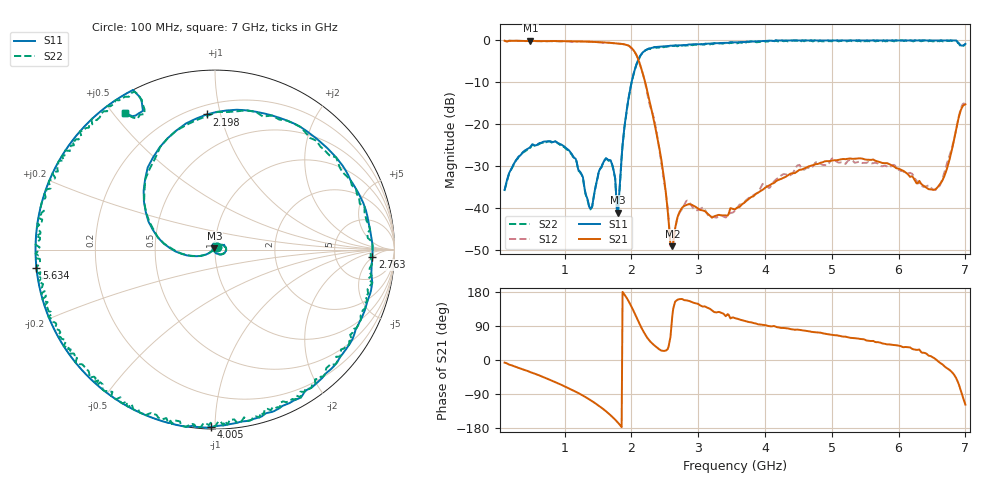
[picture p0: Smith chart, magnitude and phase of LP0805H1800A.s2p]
!	AVX	THIN	FILM	OPERATION
!	LP0805	High	Performance	Low	Pass	Filter	P/N	LP0805H1800ASTR
!	November	"13,"	2016
!Instrument:	"HEWLETT PACKARD,8720ES,US39172150,7.62 "
#	MHz	S	dB	R	50
!	Frq	S11(dB)	S11(deg)	S21(dB)	S21(deg)	S12(dB)	S12(deg)	S22(dB)	S22(deg)
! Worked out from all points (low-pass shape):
!   501 points, 100 MHz to 7 GHz, reference 50 ohm
!   highest |S21| = -0.04 dB at 486.4 MHz (marker M1); lowest = -49.2 dB at 2.612 GHz (marker M2)
!   |S21| within 3 dB of the highest: start of sweep to 2.06 GHz
!   lowest |S11| = -41.1 dB at 1.797 GHz (marker M3), VSWR 1.02, Z = 49.6 + j0.788 ohm
!   |S11| at or under -10 dB: start of sweep to 2.001 GHz
!   |S22| runs from -41.2 to 0.0 dB; largest |S21 - S12| = 0.063
!   S11 on the Smith chart (normalised r, x): 100 MHz: 1.02, +0.03; 2.198 GHz: 0.26, +0.91; 2.763 GHz: 14, -5; 4.005 GHz: 0.01, -0.98; 5.634 GHz: 0.00, -0.05; 7 GHz: 0.06, +0.54
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100  -35.75 54.8  -0.06 -6.9  -0.08 -6.6  -35.75 54.8
486.4  -25.42 26.5  -0.04 -32.1  -0.04 -31.5  -25.62 26.3
969.4  -25.07 -20.7  -0.17 -67.2  -0.22 -66.5  -25.07 -20.8
1259.2  -32.23 -66.5  -0.27 -92.6  -0.25 -92.4  -32.23 -66.6
1383.4  -40.19 -140.5  -0.30 -105.7  -0.34 -105.5  -40.39 -140.6
1535.2  -30.58 115.4  -0.42 -123.8  -0.46 -123.8  -30.58 115.4
1659.4  -28.57 89.6  -0.53 -141.4  -0.56 -141.5  -28.77 89.4
1797.4  -41.12 115.4  -0.71 -165.3  -0.74 -165.4  -41.22 115.3
1963  -13.12 -177.3  -1.29 153.3  -1.29 152.8  -13.32 -177.4
2073.4  -5.75 140.4  -3.46 113.1  -3.44 114.7  -5.85 140.4
2197.6  -2.45 93.6  -9.51 69.6  -9.69 67.9  -2.55 93.5
2404.6  -1.51 44.5  -24.66 29.6  -24.79 25.2  -1.71 44.3
2611.6  -1.22 14.3  -49.16 117.3  -48.60 115.2  -1.32 14.1
2763.4  -1.13 -2.6  -39.89 160.4  -40.12 162.1  -1.23 -2.9
3550  -0.44 -64.1  -40.39 110.4  -40.71 117.2  -0.54 -64.1
4005.4  -0.11 -91.2  -35.15 91.9  -34.44 88.3  -0.31 -91.4
4709.2  0.00 -129.8  -29.84 74.0  -30.21 75.4  -0.20 -129.8
5633.8  0.00 -174.2  -28.58 49.0  -29.26 54.4  0.00 -174.3
5854.6  0.00 174.4  -29.50 41.3  -30.28 43.3  -0.20 174.2
6572.2  0.00 136.9  -35.26 -0.6  -35.46 -5.5  -0.10 136.8
6848.2  0.00 118.3  -22.33 -43.9  -22.28 -43.5  -0.10 118.2
7000  -0.82 123.3  -15.27 -117.8  -15.23 -119.2  -0.82 123.3
